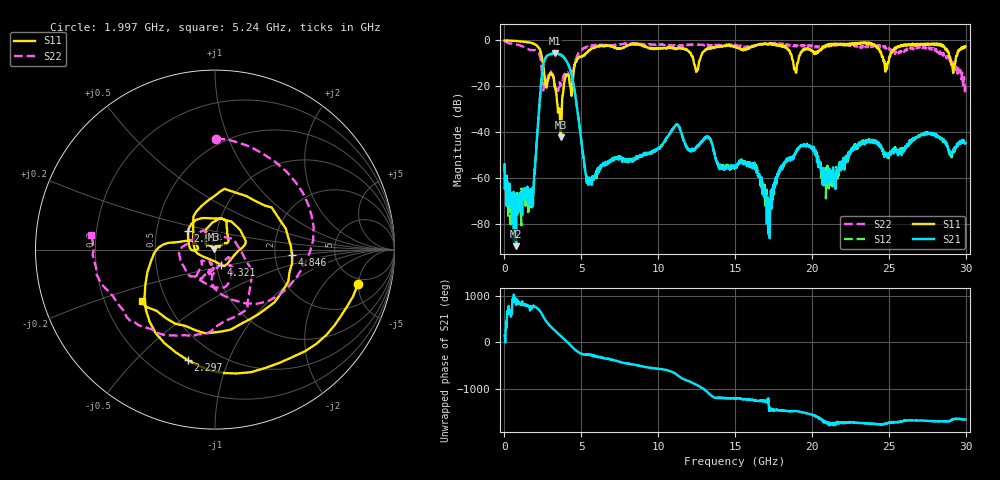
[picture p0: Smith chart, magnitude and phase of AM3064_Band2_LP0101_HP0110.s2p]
# Hz S DB R 50.0
!freq dBS11 angS11 dBS21 angS21 dBS12 angS12 dBS22 angS22
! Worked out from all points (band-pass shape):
!   1600 points, 10 MHz to 29.98 GHz, reference 50 ohm
!   highest |S21| = -5.56 dB at 3.271 GHz (marker M1); lowest = -89.5 dB at 759.8 MHz (marker M2)
!   |S21| within 3 dB of the highest: 2.607 GHz to 3.992 GHz (1.385 GHz wide, 42 % of centre)
!   lowest |S11| = -42.1 dB at 3.665 GHz (marker M3), VSWR 1.02, Z = 49.3 + j0.376 ohm
!   |S11| at or under -10 dB: 2.501 GHz to 4.595 GHz (2.094 GHz wide, 59 % of centre); 12.33 GHz to 12.64 GHz (315.3 MHz wide, 2.53 % of centre); 18.8 GHz to 19.05 GHz (251.3 MHz wide, 1.33 % of centre)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
!   |S22| runs from -23.2 to -0.2 dB; largest |S21 - S12| = 0.016
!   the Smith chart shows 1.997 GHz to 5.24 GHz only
!   S11 on the Smith chart (normalised r, x): 1.997 GHz: 4.15, -4.89; 2.297 GHz: 0.35, -0.72; 2.934 GHz: 0.72, +0.16; 4.321 GHz: 1.05, -0.18; 4.846 GHz: 2.49, -0.18; 5.24 GHz: 0.36, -0.28
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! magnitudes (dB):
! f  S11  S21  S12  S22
! 10 MHz  0.0  -54.1  -53.4  -0.2
! 759.8 MHz  -0.3  -89.5  -73.2  -1.8
! 1.734 GHz  -1.1  -64.9  -66.0  -4.2
! 1.997 GHz  -1.7  -54.7  -54.1  -4.2
! 2.297 GHz  -3.9  -26.0  -25.9  -6.7
! 2.934 GHz  -14.8  -6.2  -6.2  -13.5
! 3.271 GHz  -19.6  -5.6  -5.6  -20.3
! 3.665 GHz  -42.1  -6.5  -6.2  -19.4
! 4.321 GHz  -20.9  -13.8  -13.7  -21.1
! 4.846 GHz  -7.3  -35.4  -35.3  -5.1
! 5.015 GHz  -7.3  -44.3  -44.3  -4.1
! 5.24 GHz  -6.0  -55.4  -57.4  -3.1
! 10 GHz  -3.5  -46.9  -47.1  -1.9
! 11.24 GHz  -3.7  -36.6  -36.7  -2.6
! 15 GHz  -2.7  -54.9  -54.8  -2.0
! 16.3 GHz  -2.2  -55.5  -55.9  -2.2
! 17.22 GHz  -1.3  -82.6  -73.6  -1.6
! 18.17 GHz  -2.4  -53.8  -54.8  -2.2
! 19.99 GHz  -4.3  -46.7  -46.6  -2.2
! 21.06 GHz  -2.0  -58.7  -62.3  -2.0
! 25 GHz  -9.1  -50.2  -48.6  -3.2
! 29.98 GHz  -2.6  -44.7  -45.2  -20.2
